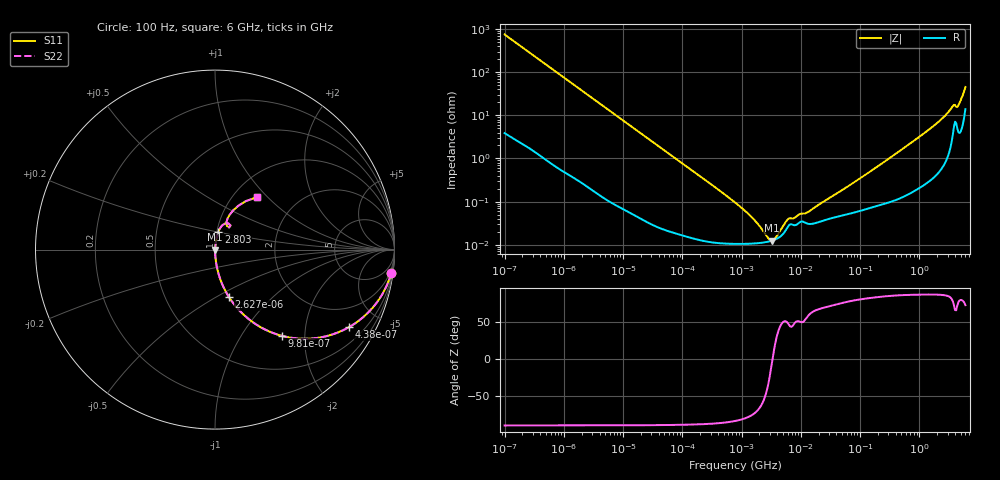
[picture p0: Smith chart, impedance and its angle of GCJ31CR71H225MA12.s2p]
!Murata Part Number: GCJ31CR71H225MA12
!These Parameters are Measured in Series Mode Connection
!Data Generated on Mar 13, 2026
!  o--ll--o
!Port1  Port2
!  o------o
!Operation Temp=25[degC], DC Bias Voltage=0[V]
!Freq. Start=100[Hz] Stop=6[GHz] 401[Steps]
# Hz S RI R 50
!Freq.(Hz) S11(Real) S11(Imag) S21(Real) S21(Imag) S12(Real) S12(Imag) S22(Real) S22(Imag)
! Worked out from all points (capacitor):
!   401 points, 100 Hz to 6 GHz, reference 50 ohm
!   read as one part in series: C = 2.12 uF near 109 Hz
!   lowest |Z| = 12.5 mohm at 3.246 MHz (marker M1)
!   series resonance near 3.339 MHz, so ESL is about 1.1 nH
!   S11 on the Smith chart (normalised r, x): 100 Hz: 1, -15; 438 Hz: 1.02, -3.44; 981 Hz: 1.01, -1.54; 2.627 kHz: 1.00, -0.58; 2.803 GHz: 1.02, +0.20; 6 GHz: 1.28, +0.87
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100  0.9818 -0.131  0.0182 0.131  0.0182 0.131  0.9818 -0.131
224  0.9171 -0.2729  0.0829 0.2729  0.0829 0.2729  0.9171 -0.2729
438  0.7458 -0.4324  0.2542 0.4324  0.2542 0.4324  0.7458 -0.4324
656  0.5692 -0.4921  0.4308 0.4921  0.4308 0.4921  0.5692 -0.4921
981  0.373 -0.4804  0.627 0.4804  0.627 0.4804  0.373 -0.4804
2008  0.1264 -0.3288  0.8736 0.3288  0.8736 0.3288  0.1264 -0.3288
2627  0.0786 -0.2655  0.9214 0.2655  0.9214 0.2655  0.0786 -0.2655
8047  0.00966 -0.0937  0.9903 0.0937  0.9903 0.0937  0.00966 -0.0937
40335  0.00061 -0.019  0.9994 0.019  0.9994 0.019  0.00061 -0.019
774597  0.000106 -0.000952  0.9999 0.000952  0.9999 0.000952  0.000106 -0.000952
1516199  0.000107 -0.000409  0.9999 0.000409  0.9999 0.000409  0.000107 -0.000409
2837864  0.000118 -7.74e-05  0.9999 7.74e-05  0.9999 7.74e-05  0.000118 -7.74e-05
3245845  0.000124 -1.34e-05  0.9999 1.34e-05  0.9999 1.34e-05  0.000124 -1.34e-05
3712478  0.000133 5.13e-05  0.9999 -5.13e-05  0.9999 -5.13e-05  0.000133 5.13e-05
6075234  0.000263 0.000288  0.9997 -0.000288  0.9997 -0.000288  0.000263 0.000288
1.555665e7  0.000306 0.000592  0.9997 -0.000592  0.9997 -0.000592  0.000306 0.000592
3.124326e8  0.00106 0.01  0.9989 -0.01  0.9989 -0.01  0.00106 0.01
1.369159e9  0.00463 0.0434  0.9954 -0.0434  0.9954 -0.0434  0.00463 0.0434
2.802721e9  0.0185 0.099  0.9815 -0.099  0.9815 -0.099  0.0185 0.099
3.666503e9  0.0557 0.1452  0.9443 -0.1452  0.9443 -0.1452  0.0557 0.1452
4.586474e9  0.0635 0.1515  0.9365 -0.1515  0.9365 -0.1515  0.0635 0.1515
6e9  0.2337 0.292  0.7663 -0.292  0.7663 -0.292  0.2337 0.292
